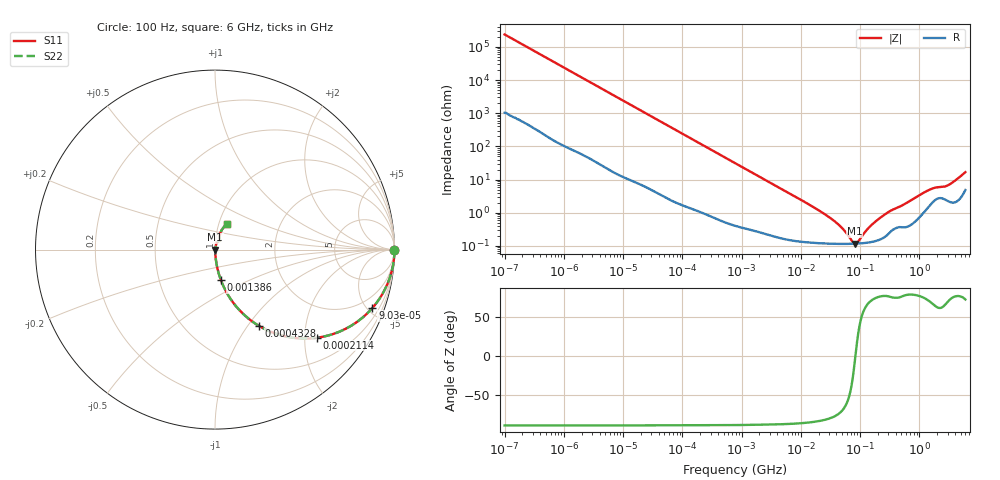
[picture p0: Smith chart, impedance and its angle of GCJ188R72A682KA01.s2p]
!Murata Part Number: GCJ188R72A682KA01
!These Parameters are Measured in Series Mode Connection
!Data Generated on Mar 13, 2026
!  o--ll--o
!Port1  Port2
!  o------o
!Operation Temp=25[degC], DC Bias Voltage=0[V]
!Freq. Start=100[Hz] Stop=6[GHz] 401[Steps]
# Hz S RI R 50
!Freq.(Hz) S11(Real) S11(Imag) S21(Real) S21(Imag) S12(Real) S12(Imag) S22(Real) S22(Imag)
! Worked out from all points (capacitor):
!   401 points, 100 Hz to 6 GHz, reference 50 ohm
!   read as one part in series: C = 6.69 nF near 109 Hz
!   lowest |Z| = 118 mohm at 81.54 MHz (marker M1)
!   series resonance near 83.48 MHz, so ESL is about 540 pH
!   S11 on the Smith chart (normalised r, x): 100 Hz: open; 90.3 kHz: 1.04, -5.38; 211.4 kHz: 1.02, -2.30; 432.8 kHz: 1.01, -1.13; 1.386 MHz: 1.01, -0.36; 6 GHz: 1.10, +0.32
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100  1 -0.000421  2e-06 0.000421  2e-06 0.000421  1 -0.000421
2008  0.9999 -0.00838  0.000111 0.00838  0.000111 0.00838  0.9999 -0.00838
12592  0.997 -0.0521  0.00299 0.0521  0.00299 0.0521  0.997 -0.0521
40335  0.9721 -0.1618  0.0279 0.1618  0.0279 0.1618  0.9721 -0.1618
90302  0.8768 -0.3254  0.1232 0.3254  0.1232 0.3254  0.8768 -0.3254
135116  0.7623 -0.4219  0.2377 0.4219  0.2377 0.4219  0.7623 -0.4219
211427  0.5698 -0.4907  0.4302 0.4907  0.4302 0.4907  0.5698 -0.4907
432798  0.2443 -0.4245  0.7557 0.4245  0.7557 0.4245  0.2443 -0.4245
774597  0.0941 -0.2856  0.9059 0.2856  0.9059 0.2856  0.0941 -0.2856
1386327  0.0333 -0.1711  0.9667 0.1711  0.9667 0.1711  0.0333 -0.1711
3712478  0.0063 -0.0663  0.9937 0.0663  0.9937 0.0663  0.0063 -0.0663
1.555665e7  0.00149 -0.0155  0.9985 0.0155  0.9985 0.0155  0.00149 -0.0155
3.983537e7  0.00118 -0.00488  0.9988 0.00488  0.9988 0.00488  0.00118 -0.00488
7.455971e7  0.00116 -0.000683  0.9988 0.000683  0.9988 0.000683  0.00116 -0.000683
8.154455e7  0.00117 -0.00014  0.9988 0.00014  0.9988 0.00014  0.00117 -0.00014
9.326766e7  0.00118 0.000674  0.9988 -0.000674  0.9988 -0.000674  0.00118 0.000674
1.275994e8  0.00125 0.00265  0.9988 -0.00265  0.9988 -0.00265  0.00125 0.00265
1.596157e8  0.00134 0.00422  0.9987 -0.00422  0.9987 -0.00422  0.00134 0.00422
3.124326e8  0.00257 0.0106  0.9974 -0.0106  0.9974 -0.0106  0.00257 0.0106
1.497423e9  0.0183 0.0455  0.9817 -0.0455  0.9817 -0.0455  0.0183 0.0455
3.065283e9  0.0257 0.061  0.9743 -0.061  0.9743 -0.061  0.0257 0.061
6e9  0.0683 0.1431  0.9317 -0.1431  0.9317 -0.1431  0.0683 0.1431
